// TwinCAT 3 PLC project PLC1
// ProgramVersion: 3.1.4022.7
// libraries:
//   Tc2_Standard, * (Beckhoff Automation GmbH)
//   Tc2_System, * (Beckhoff Automation GmbH)
//   Tc2_Utilities, * (Beckhoff Automation GmbH)
//   Tc3_Module, * (Beckhoff Automation GmbH)
// project tree:
//   / PlcTask.TcTTO
//   POUs/ MAIN.TcPOU, TimeGet.TcPOU
// real-time tasks:
//   TASK PlcTask: cycle T#22074.5us, priority 20, ADS port 350

CONFIGURATION PLC1
    RESOURCE PLC ON TwinCAT3
        TASK PlcTask(INTERVAL := T#22074.5us, PRIORITY := 20);
        PROGRAM MAIN WITH PlcTask : MAIN;
    END_RESOURCE
END_CONFIGURATION

// ---- POUs/MAIN.TcPOU
PROGRAM MAIN
VAR
END_VAR

TimeGet();

END_PROGRAM

// ---- POUs/TimeGet.TcPOU
PROGRAM TimeGet
//需要用到Tc2_System库和Tc2_Utilities库
VAR
	GETSYSTEMTIME: GETSYSTEMTIME;
	timeAsFileTime: T_FILETIME;
	timeAsSystemTime: TIMESTRUCT;	
	Temp1 		: T_ULARGE_INTEGER;
	Remainder: T_ULARGE_INTEGER;	//余数
	// UTC小于1ms的部分,单位ms
	ms1: LREAL;
	
	FB_LocalSystemTime:FB_LocalSystemTime;
	benable: BOOL;
	local_systemtime: Tc2_Utilities.TIMESTRUCT;
END_VAR

FB_LocalSystemTime(
	sNetID:='' , 
	bEnable:=benable , 
	dwCycle:= , 
	dwOpt:= , 
	tTimeout:= , 
	bValid=> , 
	systemTime=>local_systemtime , 
	tzID=> );
//获取UTC时间，格林尼治时间，伦敦时间，北京时间需要在这个时间上加8
GETSYSTEMTIME(
			timeLoDW=>timeAsFileTime.dwLowDateTime , 
			timeHiDW=>timeAsFileTime.dwHighDateTime );


//由于文件时间是以100ns为单位的64位无符号长整型，所以除以10000（16#2710）的余数就是小于ms的数值部分
Temp1 := UInt64Div64Ex( ULARGE_INTEGER( timeAsFileTime.dwHighDateTime, timeAsFileTime.dwLowDateTime ),
						ULARGE_INTEGER( 16#0, 16#2710 ),
						Remainder );
						
//小于1ms的时间转换成以ms为单位表示						
ms1:=UINT64_TO_LREAL(in:=ULARGE_INTEGER( Remainder.dwHighPart, Remainder.dwLowPart ))/10000.0;

END_PROGRAM
